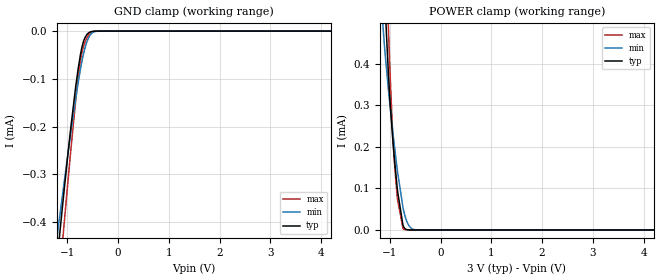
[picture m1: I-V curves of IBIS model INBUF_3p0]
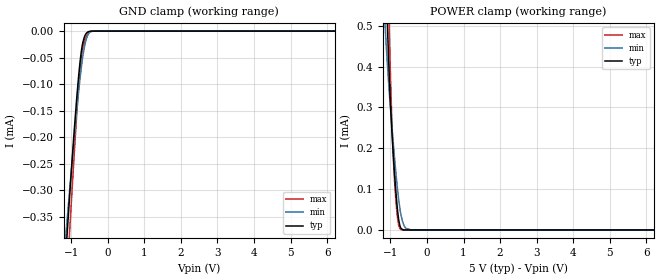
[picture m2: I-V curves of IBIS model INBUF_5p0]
|Texas Instruments Incorporated
| Marketing part#   Digital Voltage Range   Package-type   #pins
| DAC8562T   2.7V  -  5.5V   VSSOP/WSON   10
[IBIS Ver]   4.1
[File name]   dac8562t.ibs
[File Rev]   1.0
[Date]   05/13/2015
[Source]
| Texas Instruments Incorporated.
| 12500 TI Blvd
| Dallas, TX -75243
[Notes]   Revision History:
| Rev 1.0: 05/13/2015
| - Initial version of the model
| - Model generated from simulations in TISPICE
| - C_comp although listed in numerical order of value are
|   obtained from varying PVT conditions. For PVT conditions for
|   each specific value refer the buffer description under
|   respective [Model]. IBIS model user is responsible for using
|   appropriate C_comp to simulate for Signal Integrity.
| - Warnings regarding combined Non-monotonicity of various models have been
|   reviewd and considered minor and can be ignored.
| - Model names with a trailing _1p8 contain the model for
|   1.8V operation. Model names with a trailing _3p3 contain the model
|   for 3.3V operation.
[Disclaimer]
| This model is designed as an aid for customers of Texas Instruments.
| TI and its licensors and suppliers make no warranties, either expressed
| or implied, with respect to this  model, including the warranties of
| merchantability or fitness for a particular purpose. The model is
| provided solely on an "as is" basis. The entire risk as to its quality
| and performance is with the customer.
[Copyright]
 (C) Copyright 2015 Texas Instruments Incorporated.All rights reserved.
|   Device
[Component]   DAC8562T
[Manufacturer]   TI
[Package]   |VSSOP/WSON   10
| variable   typ   min   max
R_pkg   0.0712   0.0262   0.1046
L_pkg   0.9785nH   0.5979nH   1.4931nH
C_pkg   0.3322pF   0.3071pF   0.4589pF
[Pin]  signal_name   model_name   R_pin   L_pin   C_pin
1   VOUTA   NC   NA   NA   NA
2   VOUTB   NC   NA   NA   NA
3   GND   GND   NA   NA   NA
4   LDACB   INBUF   NA   NA   NA
5   CLRB   INBUF   NA   NA   NA
6   SYNCB   INBUF   NA   NA   NA
7   SCLK   INBUF   NA   NA   NA
8   DIN   INBUF   NA   NA   NA
9   AVDD   POWER   NA   NA   NA
10   VREFIN/VREFOUT   NC   NA   NA   NA
|   Model Selectors
[Model Selector]  INBUF
INBUF_3p0  input buffer at 3.0V operation.
INBUF_5p0  input buffer at 5.0V operation.
| Models and submodels in the file (2): INBUF_3p0 (Input), INBUF_5p0 (Input)
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|   Model
[Model]   INBUF_3p0
Model_type   Input
Vinl = 0.9
Vinh = 2.1
|   typ   min   max
C_comp   0.236pF   0.206pF   0.287pF
[Voltage Range]   3   2.7   3.3
[Temperature Range]   27   130   -40
[Power Clamp Reference]   3   2.7   3.3
[GND Clamp Reference]   0   0   0
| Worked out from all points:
|   POWER clamp passes 1 mA (typ) near -1.24 V on its own axis
[GND Clamp]
|   Voltage   I(typ)   I(min)   I(max)
-3V       -2.518mA   -1.982mA   -3.142mA
-1.218V   -498uA     -444.1uA   -593.4uA
-1.137V   -411.1uA   -377.3uA   -493uA
-1.083V   -354.2uA   -333.3uA   -427.5uA
-939mV    -209.3uA   -219.1uA   -258.2uA
-840mV    -120.4uA   -145.2uA   -149.7uA
-786mV    -78.41uA   -107.8uA   -97.07uA
-741mV    -48.97uA   -79.41uA   -61.42uA
-660mV    -15.61uA   -38.3uA    -25.55uA
-552mV    -2.025uA   -8.677uA   -4.521uA
-336mV    -1.716nA   -41.15nA   -547.1pA
6V        0A         0A         0A
[POWER Clamp]
|   Voltage   I(typ)   I(min)   I(max)
-3V       7.62mA     5.81mA     9.429mA
-1.146V   693.3uA    507.2uA    943.2uA
-1.092V   534.9uA    422uA      725.2uA
-1.029V   376.9uA    338.1uA    488.6uA
-948mV    226.5uA    243.4uA    241.8uA
-912mV    173.8uA    204.3uA    165uA
-849mV    94.18uA    140.5uA    73.39uA
-741mV    11.09uA    53.76uA    3.579uA
-714mV    4.743uA    39.14uA    1.15uA
-615mV    154.2nA    8.889uA    19.28nA
-471mV    0A         252.6nA    0A
6V        0A         0A         0A
|   Model
[Model]   INBUF_5p0
Model_type   Input
Vinl = 1.5
Vinh = 3.5
|   typ   min   max
C_comp   0.236pF   0.206pF   0.287pF
[Voltage Range]   5   4.5   5.5
[Temperature Range]   27   130   -40
[Power Clamp Reference]   5   4.5   5.5
[GND Clamp Reference]   0   0   0
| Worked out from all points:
|   GND clamp passes 1 mA (typ) near -1.67 V on its own axis
|   POWER clamp passes 1 mA (typ) near -1.24 V on its own axis
[GND Clamp]
|   Voltage   I(typ)   I(min)   I(max)
-5V       -4.827mA   -3.743mA   -6.082mA
-1.235V   -516.4uA   -458.2uA   -614.8uA
-1.13V    -403.6uA   -371.6uA   -484.5uA
-1.115V   -387.8uA   -359.4uA   -466.2uA
-1.085V   -356.3uA   -335uA     -430uA
-1.04V    -309.7uA   -298.7uA   -376.1uA
-860mV    -137.3uA   -159.7uA   -170.7uA
-755mV    -57.45uA   -87.93uA   -71.37uA
-680mV    -21.27uA   -46.96uA   -31.81uA
-605mV    -6.109uA   -19.85uA   -13.13uA
-530mV    -1.204uA   -5.699uA   -2.66uA
10V       0A         0A         0A
[POWER Clamp]
|   Voltage   I(typ)   I(min)   I(max)
-5V       15.38mA    11.95mA    18.81mA
-1.145V   690.2uA    505.5uA    939.1uA
-1.07V    475.8uA    391.2uA    639.8uA
-1.04V    401.9uA    351.9uA    528uA
-1.025V   368.1uA    333.1uA    474.6uA
-950mV    229.7uA    245.6uA    246.7uA
-890mV    144.2uA    181.3uA    128uA
-800mV    45.39uA    96.43uA    27.44uA
-710mV    4.15uA     37.25uA    969.1nA
-575mV    35.72nA    3.851uA    16.84nA
-425mV    0A         65.55nA    0A
10V       0A         0A         0A
